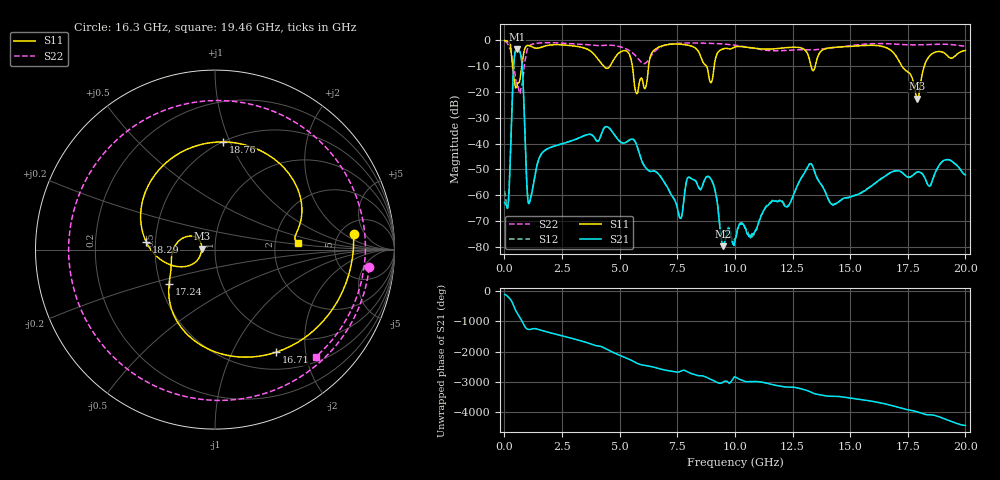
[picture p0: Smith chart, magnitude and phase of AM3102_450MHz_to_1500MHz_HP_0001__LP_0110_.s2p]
!Agilent Technologies,E8364B,MY43040894,A.07.50.67
!Agilent E8364B: A.07.50.67
!Date: Thursday, January 11, 2018 05:20:59
!Correction: S11(Full 2 Port(1,2))
!S21(Full 2 Port(1,2))
!S12(Full 2 Port(1,2))
!S22(Full 2 Port(1,2))
!S2P File: Measurements: S11, S21, S12, S22:
# Hz S  dB  R 50
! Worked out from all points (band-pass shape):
!   1601 points, 10 MHz to 20 GHz, reference 50 ohm
!   highest |S21| = -3.44 dB at 547.2 MHz (marker M1); lowest = -79.8 dB at 9.493 GHz (marker M2)
!   |S21| within 3 dB of the highest: 434.8 MHz to 727.4 MHz (292.7 MHz wide, 50.4 % of centre)
!   lowest |S11| = -22.6 dB at 17.91 GHz (marker M3), VSWR 1.16, Z = 43.1 + j0.482 ohm
!   |S11| at or under -10 dB: 350.1 MHz to 753.5 MHz (403.4 MHz wide, 73.1 % of centre); 5.553 GHz to 6.256 GHz (703.1 MHz wide, 11.9 % of centre); 17.24 GHz to 18.22 GHz (971.7 MHz wide, 5.48 % of centre)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
!   |S22| runs from -20.6 to -0.4 dB; largest |S21 - S12| = 0.0029
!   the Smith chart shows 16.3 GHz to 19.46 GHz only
!   S11 on the Smith chart (normalised r, x): 16.3 GHz: 6.61, +2.97; 16.71 GHz: 0.73, -1.51; 17.24 GHz: 0.56, -0.24; 18.29 GHz: 0.45, +0.04; 18.76 GHz: 0.50, +0.95; 19.46 GHz: 2.69, +0.24
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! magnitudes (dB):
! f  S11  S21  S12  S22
! 10 MHz  -0.1  -62.8  -58.3  -0.4
! 172.4 MHz  -0.6  -62.7  -62.8  -2.1
! 547.2 MHz  -18.0  -3.4  -3.4  -17.4
! 747.1 MHz  -10.4  -7.6  -7.6  -17.7
! 1.084 GHz  -2.1  -63.0  -62.8  -2.1
! 3.346 GHz  -2.7  -37.4  -37.4  -1.5
! 5.745 GHz  -20.7  -40.7  -40.7  -6.5
! 6.682 GHz  -2.7  -51.8  -51.7  -3.1
! 7.631 GHz  -1.5  -68.9  -68.9  -1.1
! 8.918 GHz  -16.0  -53.3  -53.2  -1.2
! 9.493 GHz  -3.3  -79.8  -79.1  -1.4
! 10.01 GHz  -2.5  -77.8  -77.0  -1.9
! 13.34 GHz  -11.1  -48.2  -48.2  -3.8
! 16.3 GHz  -2.2  -53.8  -54.1  -1.3
! 16.68 GHz  -3.3  -51.6  -51.6  -1.3
! 16.71 GHz  -3.5  -51.5  -51.5  -1.4
! 17.24 GHz  -9.9  -51.2  -51.1  -1.6
! 17.91 GHz  -22.6  -51.0  -51.0  -1.8
! 18.29 GHz  -8.3  -54.3  -54.2  -1.7
! 18.76 GHz  -4.4  -50.0  -49.9  -1.5
! 19.46 GHz  -6.7  -47.2  -47.2  -1.7
! 20 GHz  -4.0  -52.1  -51.9  -2.3
